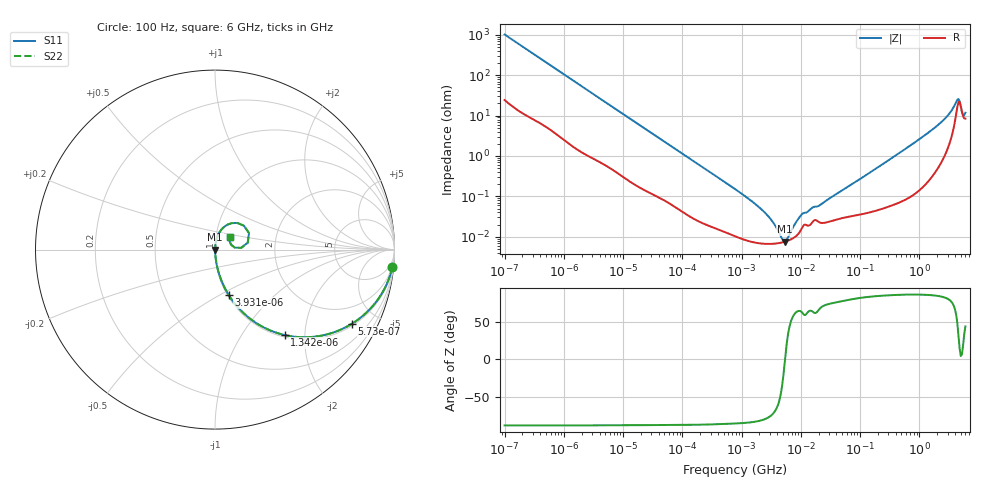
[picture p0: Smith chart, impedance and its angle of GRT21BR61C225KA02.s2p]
!Murata Part Number: GRT21BR61C225KA02
!These Parameters are Measured in Series Mode Connection
!Data Generated on Jun 19, 2026
!  o--ll--o
!Port1  Port2
!  o------o
!Operation Temp=25[degC], DC Bias Voltage=0[V]
!Freq. Start=100[Hz] Stop=6[GHz] 401[Steps]
# Hz S RI R 50
!Freq.(Hz) S11(Real) S11(Imag) S21(Real) S21(Imag) S12(Real) S12(Imag) S22(Real) S22(Imag)
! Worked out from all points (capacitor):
!   401 points, 100 Hz to 6 GHz, reference 50 ohm
!   read as one part in series: C = 1.55 uF near 109 Hz
!   lowest |Z| = 7.52 mohm at 5.312 MHz (marker M1)
!   series resonance near 5.415 MHz, so ESL is about 560 pH
!   S11 on the Smith chart (normalised r, x): 100 Hz: 1, -20; 573 Hz: 1.09, -3.66; 1.342 kHz: 1.04, -1.58; 3.931 kHz: 1.01, -0.55; 6 GHz: 1.17, +0.16
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100  0.9883 -0.0963  0.0117 0.0963  0.0117 0.0963  0.9883 -0.0963
280  0.9268 -0.2491  0.0732 0.2491  0.0732 0.2491  0.9268 -0.2491
573  0.7641 -0.4122  0.2359 0.4122  0.2359 0.4122  0.7641 -0.4122
1342  0.3875 -0.4759  0.6125 0.4759  0.6125 0.4759  0.3875 -0.4759
2008  0.2253 -0.4064  0.7747 0.4064  0.7747 0.4064  0.2253 -0.4064
3931  0.0755 -0.2514  0.9245 0.2514  0.9245 0.2514  0.0755 -0.2514
11009  0.0125 -0.0982  0.9875 0.0982  0.9875 0.0982  0.0125 -0.0982
40335  0.00171 -0.0277  0.9983 0.0277  0.9983 0.0277  0.00171 -0.0277
774597  0.000105 -0.00151  0.9999 0.00151  0.9999 0.00151  0.000105 -0.00151
2268635  6.75e-05 -0.000442  0.9999 0.000442  0.9999 0.000442  6.75e-05 -0.000442
4643984  7.12e-05 -6.96e-05  0.9999 6.96e-05  0.9999 6.96e-05  7.12e-05 -6.96e-05
5311619  7.47e-05 -8.6e-06  0.9999 8.6e-06  0.9999 8.6e-06  7.47e-05 -8.6e-06
6353432  8.19e-05 7.31e-05  0.9999 -7.31e-05  0.9999 -7.31e-05  8.19e-05 7.31e-05
9941735  0.000143 0.0003  0.9999 -0.0003  0.9999 -0.0003  0.000143 0.0003
1.555665e7  0.000225 0.000471  0.9998 -0.000471  0.9998 -0.000471  0.000225 0.000471
3.124326e8  0.000629 0.00807  0.9994 -0.00807  0.9994 -0.00807  0.000629 0.00807
1.95892e9  0.00733 0.0539  0.9927 -0.0539  0.9927 -0.0539  0.00733 0.0539
3.352442e9  0.0365 0.1123  0.9635 -0.1123  0.9635 -0.1123  0.0365 0.1123
4.193612e9  0.1236 0.1486  0.8764 -0.1486  0.8764 -0.1486  0.1236 0.1486
4.586474e9  0.1897 0.0917  0.8103 -0.0917  0.8103 -0.0917  0.1897 0.0917
5.486059e9  0.089 0.0277  0.911 -0.0277  0.911 -0.0277  0.089 0.0277
6e9  0.083 0.0693  0.917 -0.0693  0.917 -0.0693  0.083 0.0693
